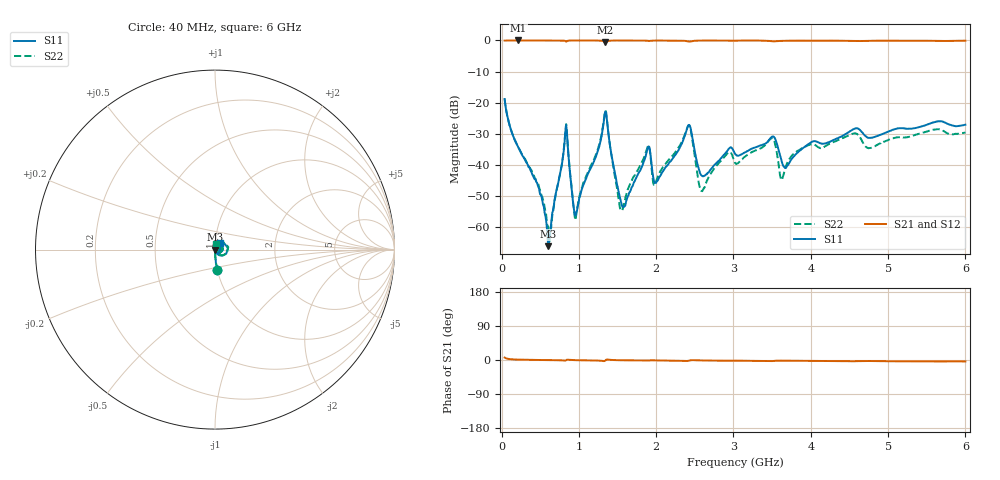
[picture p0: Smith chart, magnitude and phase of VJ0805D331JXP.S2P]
! VJ0805D331JXP
! DATE 03/14/2022  09:42
! CAPACITORS MOUNTED IN SERIES ON 25 MIL THICK MICROSTRIP SUBSTRATE
# GHz  S  MA  R  50.00
!  FREQ  S11M  S11A  S21M  S21A  S12M  S12A  S22M  S22A
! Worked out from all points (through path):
!   600 points, 40 MHz to 6 GHz, reference 50 ohm
!   highest |S21| = 0.00 dB at 219.1 MHz (marker M1); lowest = -0.7 dB at 1.343 GHz (marker M2)
!   lowest |S11| = -66.1 dB at 607.1 MHz (marker M3), VSWR 1.00, Z = 50 - j0.0222 ohm
!   |S11| at or under -10 dB: start of sweep to end of sweep
!   |S22| runs from -65.1 to -18.7 dB; largest |S21 - S12| = 0.0033
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0.04  0.1141 -83.2  0.9939 6.5  0.9927 6.5  0.1161 -83.7
0.2191  0.01867 -88.8  1 1.0  0.9998 0.9  0.01911 -88.9
0.48775  0.004078 -86.7  0.9994 0.0  0.9997 0.1  0.004292 -85.2
0.60715  0.0004934 -26.7  0.999 -0.2  1 -0.2  0.0009912 -41.7
0.64695  0.001323 55.3  0.9994 -0.3  0.9998 -0.4  0.001125 51.4
0.82605  0.03446 41.9  0.9743 -1.7  0.9754 -1.7  0.03547 42.2
0.94545  0.001676 -20.2  0.9982 -0.4  0.9994 -0.4  0.001499 -18.3
1.035  0.003951 65.2  0.999 -0.6  0.9992 -0.7  0.004172 71.7
1.34345  0.07203 7.0  0.9274 -1.3  0.9285 -1.4  0.07547 11.1
1.5524  0.002369 -26.4  0.9981 -0.6  0.9987 -0.7  0.001844 12.7
1.88075  0.01658 50.0  0.9906 -1.6  0.9918 -1.7  0.01793 61.2
1.9703  0.005557 5.2  0.9951 -0.9  0.9965 -1.0  0.004764 33.4
2.03  0.005957 45.7  0.997 -1.2  0.9982 -1.2  0.006824 75.3
2.41805  0.04335 17.6  0.9617 -2.1  0.9627 -2.2  0.04325 31.2
2.5872  0.006751 -7.7  0.9957 -1.1  0.9971 -1.2  0.003803 23.1
2.9255  0.01715 41.4  0.9935 -2.0  0.9946 -2.0  0.01546 71.6
3.025  0.01483 21.2  0.9934 -1.7  0.9946 -1.8  0.01066 57.3
3.49265  0.02805 18.2  0.9737 -2.9  0.9748 -3.0  0.02687 47.0
3.63195  0.01054 -5.6  0.9851 -1.8  0.9871 -1.8  0.005976 61.6
4.02  0.02368 45.2  0.9904 -2.6  0.9918 -2.7  0.02156 74.8
5.015  0.03472 47.8  0.9915 -3.3  0.9926 -3.4  0.02549 81.0
6.00005  0.04426 52.3  0.9897 -3.9  0.9914 -4.0  0.03331 78.0
